FUNCTION_BLOCK FB101
TITLE =Get Object
//********************************************************************************
//* maxon motor ag
//* R&D
//* all rights reserved
//********************************************************************************
//* Summary:  Reads one object from object dictionary
//*
//* Remarks:
//*
//* Created under: STEP7 REV5.2+SP1
//********************************************************************************
//* History:
//* 25.05.2004 | ina   first release
//*
//*
//********************************************************************************
//

AUTHOR:INA
FAMILY:Utilitie
NAME:GObject
VERSION:00.01


VAR_INPUT

Read : BOOL //A rising edge start the command

  NodeID : BYTE //Adress of the maxon device

  ObjectIndex : WORD //Index

  ObjectSubIndex : BYTE //SubIndex

  Length : BYTE //Object length to read

END_VAR
VAR_OUTPUT
  Done : BOOL //Data valid flag is TRUE if data were available

  Err : BOOL //Error flag is TRUE if an

  ErrNo : DINT //Contains detailed error information

  Data : DINT //Object data

END_VAR
VAR
  xEdgeMerker : BOOL //Edge Merker

  xEdgeFlag : BOOL //Edge Flag

  xStep : INT //State variable

  xObjectIndex : DWORD
  xObjectSubIndex : DWORD
END_VAR

BEGIN

NETWORK
TITLE = Activat the service function
//

// SDO Read "Get Object"

       U    #Read
       FP   #xEdgeFlag                   // recognize a positiv edge of the Read signal
       =    #xEdgeMerker                 // and set the xEdgeMerker for one cycle to true

       L    #xStep
       L    0
       ==I
       U    #xEdgeMerker
       SPB  nstp                         // iStep = 1 -> fnc1

       L    #xStep                       // jump list
       SPL  List
       SPA  rdef
       SPA  fnc1
       SPA  fncE
List  :SPA  rdef

rdef  :NOP  0                            // redefine the done signal
       R    #Done                        // reset Done
       L    0
       T    #xStep                       // iStep = 0
       SPA  end

fnc1  :NOP  0
       L    #ObjectIndex
       T    #xObjectIndex

       L    #ObjectSubIndex
       T    #xObjectSubIndex

       CALL FC1
         NodeID:=#NodeID
         Index:=#xObjectIndex
         SubIndex:=#xObjectSubIndex
         RET_VAL:=#Done
         Err:=#Err
         ErrNo:=#ErrNo

       L    #Length
       L    1
       ==I
       SPB  one

       L    #Length
       L    2
       ==I
       SPB  two
       SPA  four

one   :NOP  0
       L    DB219.DBB10
       T    #Data

       SPA  fncE

two   :NOP  0
       L    DB219.DBW10
       T    #Data

       SPA  fncE

four  :NOP  0
       L    DB219.DBD10
       T    #Data

fncE  :NOP  0
       L    0
       T    #xStep
       SPA  end

nstp  :NOP  0
       L    #xStep
       INC            1
       T    #xStep

end   :NOP  0
END_FUNCTION_BLOCK
